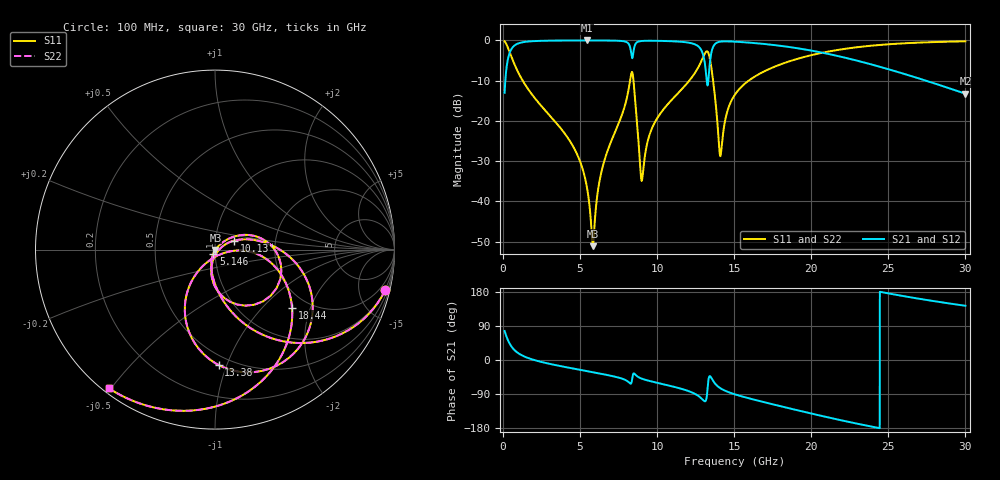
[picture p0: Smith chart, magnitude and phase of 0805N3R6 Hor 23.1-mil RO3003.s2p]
# GHz S MA R 50
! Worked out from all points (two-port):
!   3201 points, 100 MHz to 30 GHz, reference 50 ohm
!   highest |S21| = -0.02 dB at 5.445 GHz (marker M1); lowest = -13.2 dB at 30 GHz (marker M2)
!   |S21| within 3 dB of the highest: 434.7 MHz to 8.309 GHz (7.874 GHz wide, 180 % of centre); 13.52 GHz to 20.66 GHz (7.144 GHz wide, 41.8 % of centre)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
!   lowest |S11| = -51.1 dB at 5.828 GHz (marker M3), VSWR 1.01, Z = 50.2 - j0.15 ohm
!   |S11| at or under -10 dB: 1.273 GHz to 8.239 GHz (6.966 GHz wide, 146 % of centre); 8.463 GHz to 12.09 GHz (3.623 GHz wide, 35.3 % of centre); 13.63 GHz to 15.94 GHz (2.309 GHz wide, 15.6 % of centre)
!   |S22| runs from -51.1 to -0.2 dB; largest |S21 - S12| = 0
!   S11 on the Smith chart (normalised r, x): 100 MHz: 0.92, -8.38; 5.146 GHz: 0.98, -0.05; 10.13 GHz: 1.23, +0.12; 13.38 GHz: 0.43, -0.94; 18.44 GHz: 1.65, -1.51; 30 GHz: 0.02, -0.49
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0.1  0.9748 -13.4  0.223 76.5  0.223 76.5  0.9748 -13.4
0.47375  0.6766 -50.0  0.7359 39.9  0.7359 39.9  0.6766 -50.0
1.230594  0.3265 -77.7  0.9441 12.2  0.9441 12.2  0.3265 -77.7
5.089563  0.02797 -111.7  0.997 -26.6  0.997 -26.6  0.02797 -111.7
5.145625  0.02591 -111.7  0.9971 -27.1  0.9971 -27.1  0.02591 -111.7
5.444625  0.01489 -109.4  0.9971 -29.3  0.9971 -29.3  0.01489 -109.4
5.827719  0.002784 -32.5  0.997 -32.2  0.997 -32.2  0.002784 -32.5
6.444406  0.02609 45.6  0.9961 -37.0  0.9961 -37.0  0.02609 45.6
8.303812  0.3748 -12.2  0.7158 -62.0  0.7158 -62.0  0.3748 -12.2
9.004594  0.01806 -31.3  0.9825 -49.3  0.9825 -49.3  0.01806 -31.3
10.06978  0.1132 25.5  0.9861 -60.9  0.9861 -60.9  0.1132 25.5
10.12584  0.1175 25.1  0.9856 -61.4  0.9856 -61.4  0.1175 25.1
12.24687  0.3465 1.4  0.9187 -85.4  0.9187 -85.4  0.3465 1.4
12.97569  0.6148 -28.0  0.6673 -105.6  0.6673 -105.6  0.6148 -28.0
13.37747  0.6439 -88.2  0.432 -43.8  0.432 -43.8  0.6439 -88.2
13.60172  0.3475 -118.7  0.8042 -53.2  0.8042 -53.2  0.3475 -118.7
14.09694  0.03643 -64.1  0.9637 -74.4  0.9637 -74.4  0.03643 -64.1
15.05  0.2126 -4.4  0.9631 -90.7  0.9631 -90.7  0.2126 -4.4
18.44178  0.5384 -37.2  0.8334 -126.2  0.8334 -126.2  0.5384 -37.2
20.03956  0.6574 -52.4  0.7441 -141.6  0.7441 -141.6  0.6574 -52.4
25.01978  0.8942 -94.9  0.4373 175.6  0.4373 175.6  0.8942 -94.9
30  0.9731 -127.4  0.2176 143.1  0.2176 143.1  0.9731 -127.4
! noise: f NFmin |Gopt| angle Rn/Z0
0.1  0.000876  0.9305  1.229  0.002802
3.417  0.005973  0.6899  19.47  0.003644
6.743  0.01203  0.7005  36.98  0.007095
10.06  0.01994  0.7334  54.01  0.01192
13.39  0.2569  0.9697  70.66  1.281
16.7  0.02942  0.7214  84.63  0.01169
20.03  0.03444  0.7256  97.79  0.01114
23.35  0.0443  0.7587  110.6  0.01253
26.67  0.05967  0.8027  123.3  0.01475
30  0.08455  0.8509  136  0.01761
